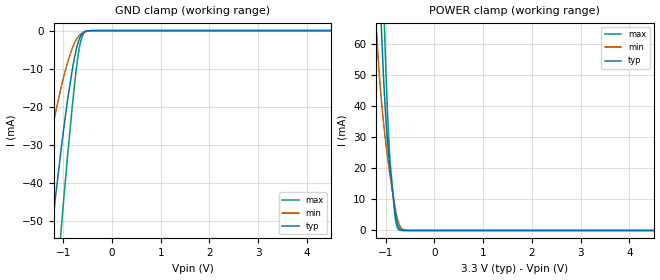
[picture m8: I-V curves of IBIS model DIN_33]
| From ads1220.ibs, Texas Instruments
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|   DIN_33 Model
[Model]   DIN_33
Model_type   Input
Vinl = .9
Vinh = 2.52
|   typ   min   max
|   (nom PVT)   (Fast PVT)   (slow PVT)
C_comp   6.455p   5.987p   6.886p
| Where   nom PVT is  Nominal Process, 3.3V, 27C
|   Fast PVT is Strong Process, 3.6V, -40C
|   Slow PVT is Weak Process, 3.0V, 125C
[Voltage Range]   3.3   3   3.6
[Temperature Range]   27   125   -40
[Power Clamp Reference]   3.3   3   3.6
[GND Clamp Reference]   0   0   0
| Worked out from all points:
|   GND clamp passes 1 mA (typ) near -0.62 V on its own axis
|   POWER clamp passes 1 mA (typ) near -0.73 V on its own axis
[GND Clamp]
|   Voltage   I(typ)   I(min)   I(max)
-3.3V     -336.7mA   -217.5mA   -424.2mA
-1.597V   -97.62mA   -52.79mA   -141.3mA
-1.241V   -53.01mA   -26.74mA   -83.07mA
-1.142V   -41.67mA   -20.52mA   -67.38mA
-1.033V   -29.98mA   -14.31mA   -50.62mA
-904.2mV  -17.58mA   -8.028mA   -31.84mA
-815.1mV  -10.27mA   -4.613mA   -19.88mA
-735.9mV  -5.129mA   -2.434mA   -10.49mA
-686.4mV  -2.81mA    -1.516mA   -5.795mA
-646.8mV  -1.522mA   -1mA       -3.081mA
-557.7mV  -238.1uA   -352.4uA   -406.3uA
6.6V      0A         0A         0A
[POWER Clamp]
|   Voltage   I(typ)   I(min)   I(max)
-3.3V     1.26A      960mA      1.562A
-1.251V   136.2mA    81.55mA    194.9mA
-1.162V   94.51mA    56.61mA    140.4mA
-1.102V   69.49mA    44.05mA    105.6mA
-1.043V   48.38mA    34.31mA    73.26mA
-1.013V   39.82mA    30.13mA    58.54mA
-953.7mV  26.65mA    22.55mA    34.06mA
-914.1mV  19.9mA     17.91mA    22.51mA
-815.1mV  6.743mA    7.81mA     5.18mA
-716.1mV  575.1uA    1.611mA    127.3uA
-518.1mV  231.2nA    8.258uA    0A
6.6V      0A         0A         0A
